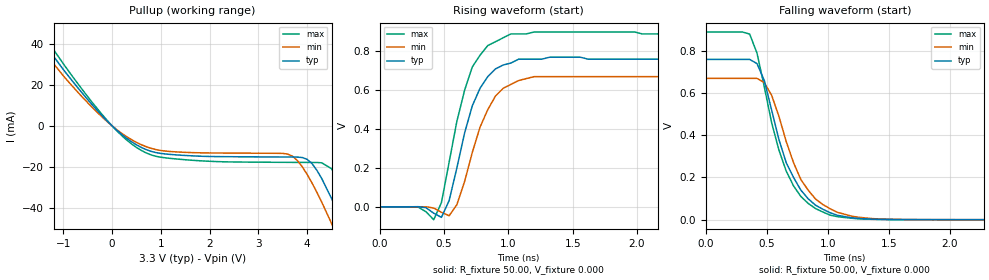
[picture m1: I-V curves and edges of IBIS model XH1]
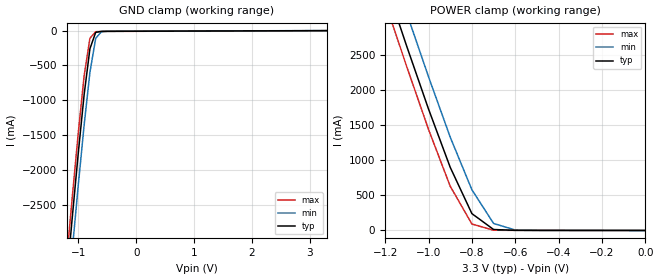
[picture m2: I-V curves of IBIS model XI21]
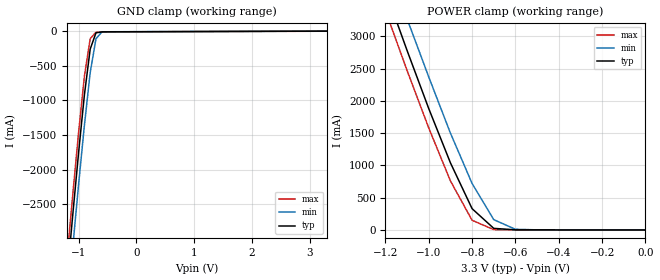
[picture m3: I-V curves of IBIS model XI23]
|   * 9db833a.ibs * IBIS 2.1 Model file
| Rev History
| Rev No.   Description
| 1.1   Initial release
| 1.2   Updated pin names, removed unused input model.
[IBIS Ver]   2.1
[Comment char]  |_char
[File name]   9db833a.ibs
|[Date]   June 12, 2006
|[File Rev]   1.0
|[Date]   May 10, 2010
|[File Rev]   1.1
|   Added Vmeas, Vref, Rref
[Date]   Aug 30, 2011
[File Rev]   1.2
|   Rename pins. #2=VDDR, #40=PD#,All OE now OE# lfp
[Source]   Originated at Integrated Circuit Systems, Inc.
[Disclaimer] (C) Copyright Integrated Circuit Systems, Inc. 2006
   All rights reserved
ICS hereby grants the user of this IBIS model a non-exclusive,
nontransferable license to use this IBIS model under the following terms.
Before using this IBIS model, the user should read this license.
If the user does not accept these terms,  the IBIS model should be
returned to ICS within 30 days.
   The user is granted this license only to use the IBIS model and
is not granted rights to sell, load, rent, lease or license the IBIS
model in whole or in part, or in modified form to anyone other than
user. User may modify the IBIS model to suit its specific
applications but rights to derivative works and such modifications
shall belong to ICS.
   This IBIS model is provided on an "AS IS" basis and ICS makes
absolutely no warranty with respect to the information contained
herein. ICS DISCLAIMS AND CUSTOMER WAIVES ALL WARRANTIES, EXPRESS
OR IMPLIED, INCLUDING WARRANTIES OF MERCHANTABILITY OR FITNESS FOR
A PARTICULAR PURPOSE. The entire risk as to quality and performance
is with the Customer. ACCORDINGLY, IN NO EVENT SHALL THE COMPANY BE
LIABLE FOR ANY DAMAGES, WHETHER IN CONTRACT OR TORT,INCLUDING ANY
LOST PROFITS OR OTHER INCIDENTAL, CONSEQUENTIAL, EXEMPLARY, OR
PUNITIVE DAMAGES ARISING OUT OF THE USE OR APPLICATION OF THE IBIS
model provided in this package. Further, ICS reserves the right to
make changes without notice to any product herein to improve
reliability, function, or design. ICS does not convey any license
under patent rights or any other intellectual property rights,
including those of third parties.
   ICS is not obligated to provide maintenance or support
for the licensed IBIS model.
|   COMPONENT: ICS9db833a
[Component]   ICS9db833a
[Manufacturer]  ICS
[Package]
| variable   typ   min   max
R_pkg   70.0m   50.0m   90.0m
L_pkg   5.1nH   3.2nH   7.0nH
C_pkg   0.70pF  0.50pF  0.90pF
[Pin]   signal_name   model_name   R_pin   L_pin   C_pin
  1   SRCDIVB   XI23
  2   VDDR   POWER
  3   VSS   GND
  4   SRC_IN   XI4
  5   SRC_IN#   XI4
  6   OE_0#   XI21
  7   OE_3#   XI21
  8   DIF_0   XH1
  9   DIF_0#   XH1
 10   GND   GND
 11   VDD   POWER
 12   DIF_1   XH1
 13   DIF_1#   XH1
 14   OE_1#   XI23
 15   OE_2#   XI23
 16   DIF_2   XH1
 17   DIF_2#   XH1
 18   GND   GND
 19   VDD   POWER
 20   DIF_3   XH1
 21   DIF_3#   XH1
 22   BYPASS#/LOBW/HGBW   XI23
 23   SCLK   XI10
 24   SDATA   XIO3
 25   GND   GND
 26   GND   GND
 27   VDD   POWER
 28   SMB_ADR   XI23
 29   DIF_4#   XH1
 30   DIF_4   XH1
 31   VDD   POWER
 32   GND   GND
 33   DIF_5#   XH1
 34   DIF_5   XH1
 35   OE_5#   XI23
 36   OE_6#   XI23
 37   DIF_6#   XH1
 38   DIF_6   XH1
 39   VDD   POWER
 40   PD#   XI24
 41   DIF_7#   XH1
 42   DIF_7   XH1
 43   OE_4#   XI21
 44   OE_7#   XI21
 45   LOCKOUT   XO1
 46   IREF   XI29
 47   GNDA   GND
 48   VDDA   POWER
|* Either 3.3V or 2.5V
|** All model are simulated with typical corner process
[Diff Pin]   inv_pin   vdiff   tdelay_typ
4   5   NA   NA
8   9   NA   NA
12   13   NA   NA
16   17   NA   NA
20   21   NA   NA
30   29   NA   NA
34   33   NA   NA
38   37   NA   NA
42   41   NA   NA
| Models and submodels in the file (9): XH1 (Open_source), XI21 (Input), XI23 (Input), XI24 (Input), XI29 (Input), XI10 (Input), XI4 (Input), XIO3 (I/O_open_drain), XO1 (Output)
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|   Model XH1
[Model]   XH1
Model_type   Open_source
Polarity   Inverting
Vmeas = 0.35V
Cref =   2.00pF
Rref =  500
Vref =   0.0V
C_comp   3.40pF   2.85pF   3.95pF
[Temperature Range]   25.00   70.00   0.000
[Voltage Range]   3.30V   3.00V   3.70V
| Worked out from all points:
|   slope of the pullup table from 0 to 0.495 V, typ, clamps not added: 53.7 ohm
|   rising waveform, R_fixture 50.00, V_fixture 0.000: 20-80 % time 196ps typ, 209ps min, 191ps max; typ from 0 V to 0.76 V
|   falling waveform, R_fixture 50.00, V_fixture 0.000: 20-80 % time 266ps typ, 276ps min, 255ps max; typ from 0.76 V to 0 V
[Pullup]
| voltage   I(typ)   I(min)   I(max)
-3.3V     120mA      110mA      120mA
-1.9V     57.97mA    52.49mA    62.98mA
-1.5V     43.73mA    39.31mA    47.78mA
-100mV    2.37mA     2.07mA     2.66mA
700mV     -11.65mA   -10.21mA   -13.27mA
3.6V      -15.27mA   -13.83mA   -17.88mA
4V        -16.4mA    -23.77mA   -17.93mA
4.3V      -25.83mA   -37.4mA    -18.11mA
4.5V      -35.53mA   -47.74mA   -20.97mA
4.7V      -46.5mA    -58.63mA   -28.65mA
5.1V      -70.24mA   -81.19mA   -50.61mA
6.6V      -160mA     -170mA     -150mA
[Ramp]
| variable   typ   min   max
dV/dt_r   0.46/0.20n   0.40/0.21n   0.53/0.19n
dV/dt_f   0.45/0.26n   0.40/0.27n   0.53/0.25n
R_load = 50.00
[Rising Waveform]
R_fixture = 50.00
V_fixture = 0.000
V_fixture_min = 0.000
V_fixture_max = 0.000
| time   V(typ)   V(min)   V(max)
0s        -370nV     -380nV     -340nV
300ps     550uV      230uV      -1.44mV
420ps     -32.86mV   -6.35mV    -66.34mV
480ps     -54.44mV   -28.27mV   21.55mV
540ps     32.24mV    -46.01mV   230mV
600ps     200mV      10.91mV    440mV
720ps     520mV      280mV      720mV
840ps     670mV      500mV      830mV
1.02ns    740mV      630mV      890mV
3ns       760mV      670mV      890mV
[Falling Waveform]
R_fixture = 50.00
V_fixture = 0.000
V_fixture_min = 0.000
V_fixture_max = 0.000
| time   V(typ)   V(min)   V(max)
0s        760mV      670mV      890mV
360ps     760mV      670mV      880mV
420ps     740mV      670mV      790mV
480ps     660mV      650mV      630mV
540ps     520mV      590mV      460mV
660ps     270mV      370mV      230mV
780ps     140mV      190mV      110mV
900ps     68.75mV    97.98mV    52.94mV
1.38ns    2.27mV     4.59mV     1.49mV
3ns       -13.74uV   -37.6uV    -15.05uV
|   Model XI21
|   Input has internal pull-up resistor
[Model]   XI21
Model_type   Input
Polarity   Inverting
Enable   Active-High
Vinl =   0.80V
Vinh =   2.00V
C_comp   3.40pF   2.85pF   3.95pF
[Temperature Range]   27.00   70.00   0.000
[Voltage Range]   3.30V   3.00V   3.70V
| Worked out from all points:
|   POWER clamp passes 1 mA (typ) near -0.39 V on its own axis
[GND_clamp]
| voltage   I(typ)   I(min)   I(max)
-3.3V     -24.07A    -24.5A     -23.8A
-1.2V     -3.56A     -4.03A     -3.27A
-1.1V     -2.64A     -3.11A     -2.35A
-1V       -1.75A     -2.21A     -1.46A
-900mV    -920mA     -1.36A     -650mA
-800mV    -260mA     -600mA     -110mA
-700mV    -25mA      -110mA     -15.24mA
-600mV    -10.97mA   -15.13mA   -11.57mA
-500mV    -9.91mA    -9.4mA     -10.9mA
3.3V      450nA      780uA      -1.03mA
[POWER_clamp]
| voltage   I(typ)   I(min)   I(max)
-3.3V     24.04A     24.47A     23.78A
-1.2V     3.54A      4.01A      3.25A
-1.1V     2.62A      3.09A      2.33A
-1V       1.73A      2.19A      1.44A
-900mV    900mA      1.33A      630mA
-800mV    240mA      580mA      92.42mA
-700mV    13.81mA    100mA      3.74mA
-600mV    1.83mA     6.31mA     1.58mA
0V        130pA      310pA      130pA
|   Model XI23
|   Input has internal pull-up resistor
[Model]   XI23
Model_type   Input
Polarity   Inverting
Enable   Active-High
Vinl =   0.80V
Vinh =   2.00V
C_comp   3.40pF   2.85pF   3.95pF
[Temperature Range]   27.00   70.00   0.000
[Voltage Range]   3.30V   3.00V   3.70V
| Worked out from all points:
|   POWER clamp passes 1 mA (typ) near -0.39 V on its own axis
[GND_clamp]
| voltage   I(typ)   I(min)   I(max)
-3.3V     -24.07A    -24.5A     -23.8A
-1.2V     -3.56A     -4.03A     -3.27A
-1.1V     -2.64A     -3.11A     -2.35A
-1V       -1.75A     -2.21A     -1.46A
-900mV    -920mA     -1.36A     -650mA
-800mV    -260mA     -600mA     -110mA
-700mV    -24.92mA   -110mA     -15.24mA
-600mV    -10.96mA   -15.13mA   -11.57mA
-500mV    -9.91mA    -9.4mA     -10.9mA
3.3V      130pA      780uA      -1.03mA
[POWER_clamp]
| voltage   I(typ)   I(min)   I(max)
-3.3V     24.22A     24.67A     23.94A
-1.2V     3.71A      4.2A       3.4A
-1.1V     2.78A      3.27A      2.47A
-1V       1.88A      2.37A      1.58A
-900mV    1.04A      1.5A       760mA
-800mV    330mA      720mA      150mA
-700mV    24.76mA    160mA      5.64mA
-600mV    2.11mA     10.91mA    1.62mA
0V        130pA      310pA      130pA
